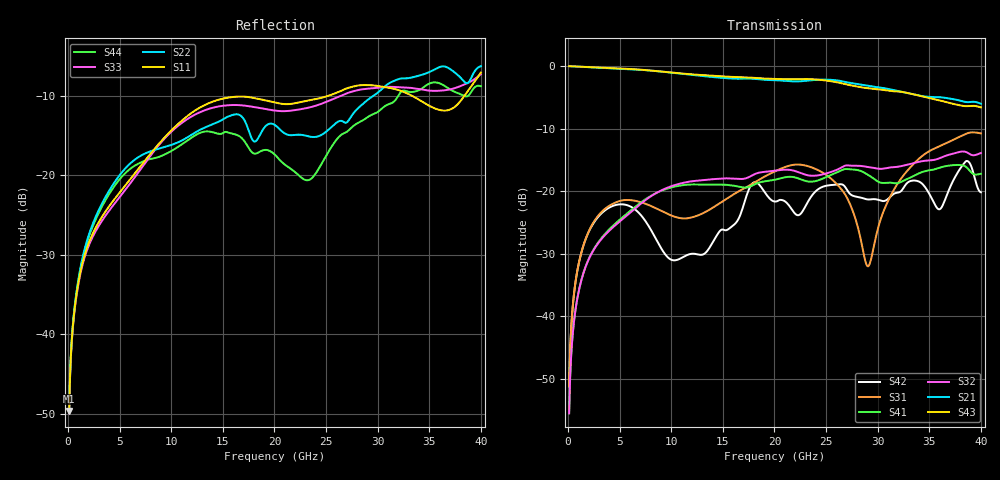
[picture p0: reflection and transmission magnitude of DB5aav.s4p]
! ADC12DJ2700AAV, ADC12DJ3200AAV, ADC08DJ3200AAV
! 144 pin AAV package
! Texas Instruments 4/21/2021
! Single-ended  S-parameters
! PORT#  PORT_NAME  NET_NAME
! PORT1:  DAxN.DIEBUMP DAxN
! PORT2:  DAxN.BGA  DAxN
! PORT3:  DAxP.DIEBUMP DAxP
! PORT4:  DAxP.BGA  DAxP
! Touchstone Ver. 1.0
! Number of ports is 4
# Hz	S	MA	R	50.000000
! SCATTERING PARAMETERS  :
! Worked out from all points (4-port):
!   400 points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, 100 MHz to 40 GHz, reference 50 ohm
!   strongest paths, dB at 100 MHz, 10.1 GHz, 20.1 GHz, 30.1 GHz, 40 GHz:
!     S43: 0.0, -1.0, -2.1, -3.7, -6.6
!     S21: 0.0, -1.1, -2.3, -3.4, -6.0
!     S32: -55.5, -19.1, -16.7, -16.4, -13.9
!     S41: -55.5, -19.4, -18.1, -18.5, -17.2
!     S31: -51.2, -23.9, -16.8, -25.5, -10.8
!     S42: -51.2, -31.0, -21.6, -21.4, -20.2
!   lowest |S11| = -49.7 dB at 100 MHz (marker M1), VSWR 1.01, Z = 50.2 + j0.288 ohm
!   |S11| at or under -10 dB: start of sweep to 25.13 GHz; 33.38 GHz to 38.39 GHz (5.007 GHz wide, 14 % of centre)
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1e8  0.003279 61.0  0.9982 -1.3  0.002763 85.0  0.001682 -97.3
     0.9982 -1.3  0.003295 59.8  0.001682 -97.3  0.002761 84.6
     0.002763 85.0  0.001682 -97.3  0.003173 61.6  0.9982 -1.3
     0.001682 -97.3  0.002761 84.6  0.9982 -1.3  0.003189 60.3
9e8  0.01943 68.3  0.9913 -11.2  0.02335 75.8  0.014 -109.5
     0.9913 -11.2  0.02018 54.9  0.01398 -109.6  0.02325 72.2
     0.02335 75.8  0.01398 -109.6  0.01894 69.0  0.9915 -10.8
     0.014 -109.5  0.02325 72.2  0.9915 -10.8  0.01972 54.8
3.1e9  0.05244 59.2  0.9705 -37.4  0.06645 49.6  0.04091 -145.0
       0.9705 -37.4  0.06295 10.8  0.04024 -144.8  0.06491 37.2
       0.06645 49.6  0.04024 -144.8  0.04962 62.2  0.9715 -36.1
       0.04091 -145.0  0.06491 37.2  0.9715 -36.1  0.0604 9.8
1.5e10  0.3046 -12.6  0.8043 -172.6  0.08322 42.7  0.1128 50.7
        0.8043 -172.6  0.2254 -118.9  0.1264 57.9  0.04944 34.7
        0.08322 42.7  0.1264 57.9  0.2746 1.4  0.8276 -166.5
        0.1128 50.7  0.04944 34.7  0.8276 -166.5  0.1845 -126.4
2.36e10  0.2994 -59.6  0.771 93.3  0.155 1.6  0.1192 -46.5
         0.771 93.3  0.1748 88.5  0.133 -42.4  0.09173 -15.3
         0.155 1.6  0.133 -42.4  0.2702 -38.0  0.7854 99.6
         0.1192 -46.5  0.09173 -15.3  0.7854 99.6  0.09588 58.6
2.94e10  0.3699 -97.9  0.6877 19.7  0.02963 46.4  0.1299 -126.3
         0.6877 19.7  0.3112 -44.8  0.1547 -107.2  0.08627 175.7
         0.02963 46.4  0.1547 -107.2  0.3537 -76.7  0.6599 32.9
         0.1299 -126.3  0.08627 175.7  0.6599 32.9  0.2407 -62.1
4e10  0.4446 32.3  0.5002 -112.1  0.2898 -14.8  0.138 98.1
      0.5002 -112.1  0.4878 -106.1  0.202 123.9  0.09815 57.8
      0.2898 -14.8  0.202 123.9  0.434 99.8  0.4678 -85.2
      0.138 98.1  0.09815 57.8  0.4678 -85.2  0.3647 -116.4
